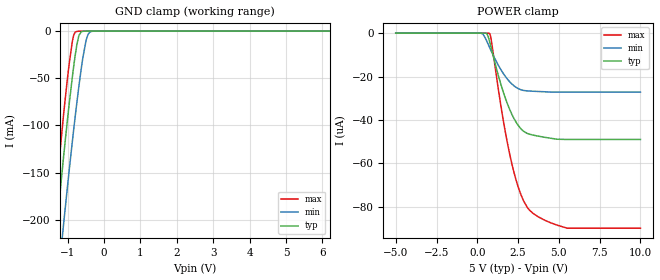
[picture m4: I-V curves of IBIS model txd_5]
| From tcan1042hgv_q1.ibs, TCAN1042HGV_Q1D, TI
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|   txd_5 Model
[Model]   txd_5
Model_type   Input
Vinl = 1.5
Vinh = 3.5
|   typ   min   max
|   (nom PVT)   (fast PVT)   (slow PVT)
C_comp   2.287e-12   2.118e-12   2.744e-12
| Where nom  PVT is Nominal Process, 5V, 27C
|   Fast PVT is Strong Process,  5.5V, -55C
|   Slow PVT is Weak Process,   4.5V, 150C
[Voltage Range]   5   4.5   5.5
|Junction Temperature
[Temperature Range]   27   150   -55
[Power Clamp Reference]   5   4.5   5.5
[GND Clamp Reference]   0   0   0
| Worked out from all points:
|   GND clamp passes 1 mA (typ) near -0.63 V on its own axis
[GND Clamp]
|   Voltage   I(typ)   I(min)   I(max)
-5V       -1.891A    -1.922A    -1.879A
-1.522V   -297.1mA   -366.4mA   -254.9mA
-1.373V   -235.5mA   -306.1mA   -191.9mA
-1.115V   -133.5mA   -205.2mA   -88.84mA
-960mV    -77.35mA   -147.7mA   -34.78mA
-875mV    -49.3mA    -117.7mA   -11.26mA
-825.5mV  -34.32mA   -100.8mA   -3.135mA
-750mV    -14.75mA   -76.11mA   -374.7uA
-630mV    -834.4uA   -40.28mA   -23.45uA
-500mV    -25.05uA   -10.77mA   -1.409uA
-329mV    -545.1nA   -243.3uA   -638.6nA
10V       0A         0A         0A
[POWER Clamp]
|   Voltage   I(typ)   I(min)   I(max)
-5V       0A         120.9nA    0A
211mV     0A         33.05nA    0A
560mV     -118.4nA   -3.349uA   0A
753mV     -3.857uA   -6.574uA   -165.8nA
890.5mV   -7.965uA   -8.838uA   -4.838uA
1.6V      -27.33uA   -18.67uA   -40.53uA
2.018V    -35.76uA   -22.68uA   -56.9uA
2.502V    -42.48uA   -25.54uA   -70.81uA
3.1V      -46.34uA   -26.65uA   -80.68uA
4.053V    -47.93uA   -27uA      -85.97uA
5.505V    -49.02uA   -27.21uA   -89.93uA
10V       -49.02uA   -27.21uA   -89.93uA
